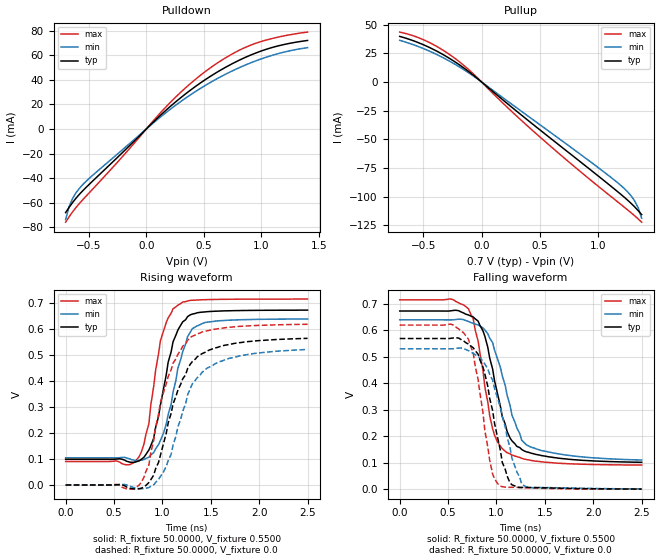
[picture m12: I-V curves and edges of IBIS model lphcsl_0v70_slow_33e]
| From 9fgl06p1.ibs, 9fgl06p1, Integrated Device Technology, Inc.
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[Model]   lphcsl_0v70_slow_33e
Model_type Output
Polarity   Inverting
Enable   Active-High
Vmeas =  0.4000V
Cref =   2.0000pF
Rref =   0.0
Vref =   0.4000V
C_comp   1.1000pF   1.0000pF   1.2000pF
[Temperature Range]   25.0000   85.0000   -40.0000
[Voltage Range]   0.7000V   0.6700V   0.7400V
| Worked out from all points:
|   slope of the pulldown table from 0 to 0.105 V, typ, clamps not added: 10.9 ohm
|   slope of the pullup table from 0 to 0.105 V, typ, clamps not added: 11.6 ohm
|   rising waveform, R_fixture 50.0000, V_fixture 0.5500: 20-80 % time 192ps typ, 209ps min, 165ps max; typ from 0.099 V to 0.672 V
|   rising waveform, R_fixture 50.0000, V_fixture 0.0: 20-80 % time 288ps typ, 300ps min, 271ps max; typ from 0 V to 0.563 V
|   falling waveform, R_fixture 50.0000, V_fixture 0.5500: 20-80 % time 218ps typ, 259ps min, 183ps max; typ from 0.672 V to 0.102 V
|   falling waveform, R_fixture 50.0000, V_fixture 0.0: 20-80 % time 190ps typ, 227ps min, 157ps max; typ from 0.568 V to 0.001 V
[Pulldown]
|Voltage   I(typ)   I(min)   I(max)
-700mV    -68.01mA   -73.7mA    -75.8mA
-670mV    -63.71mA   -63.29mA   -71.42mA
-640mV    -59.83mA   -56.58mA   -67.45mA
-580mV    -53.07mA   -48.2mA    -60.55mA
-520mV    -47.27mA   -42.3mA    -54.39mA
170mV     15.18mA    13.27mA    17.9mA
320mV     27.03mA    23.73mA    31.72mA
470mV     37.47mA    33.03mA    43.69mA
680mV     49.79mA    44.19mA    57.46mA
890mV     59.52mA    53.22mA    67.62mA
1.13V     67.27mA    60.95mA    74.47mA
1.4V      72.06mA    66.21mA    78.86mA
[Pullup]
|Voltage   I(typ)   I(min)   I(max)
-700mV    39.71mA    36.3mA     43.49mA
-580mV    35.81mA    32.37mA    40.12mA
-460mV    30.74mA    27.51mA    35.06mA
-220mV    17.02mA    14.97mA    19.97mA
-70mV     5.896mA    5.136mA    7.022mA
350mV     -29.63mA   -26.26mA   -34.41mA
770mV     -63.63mA   -57.46mA   -71.78mA
1.1V      -90.4mA    -82.71mA   -99.38mA
1.25V     -103.2mA   -95.91mA   -111.7mA
1.31V     -109mA     -103.8mA   -116.8mA
1.34V     -112.3mA   -109.8mA   -119.5mA
1.37V     -115.8mA   -118.9mA   -122.4mA
[Ramp]
| variable   typ   min   max
dV/dt_r  0.3379/0.2954n   0.3123/0.3248n   0.3703/0.2635n
dV/dt_f  0.3418/0.2381n   0.3163/0.2687n   0.3737/0.1983n
R_load = 50.0000
[Rising Waveform]
R_fixture= 50.0000
V_fixture= 0.5500
V_fixture_min= 0.5200
V_fixture_max= 0.5800
|time   V(typ)   V(min)   V(max)
0s        98.56mV    104.2mV    90.22mV
660ps     88.18mV    100.7mV    78.13mV
760ps     92.78mV    94.19mV    109.3mV
860ps     134mV      106.6mV    234.8mV
980ps     307.9mV    171.6mV    554.8mV
1.06ns    472.2mV    271.4mV    642.1mV
1.16ns    595.2mV    449.4mV    690.7mV
1.26ns    646.7mV    569.6mV    706.7mV
1.41ns    663.9mV    619.8mV    711.5mV
2.5ns     671.6mV    637.7mV    714.1mV
[Rising Waveform]
R_fixture= 50.0000
V_fixture= 0.0
V_fixture_min= 0.0
V_fixture_max= 0.0
|time   V(typ)   V(min)   V(max)
0s        0V         0V         0V
760ps     -14.65mV   -13.93mV   62.88uV
860ps     9.248mV    -10.24mV   76.78mV
960ps     86.84mV    21.5mV     271.9mV
1.01ns    157mV      49.52mV    353.9mV
1.11ns    311.2mV    152.8mV    467.7mV
1.29ns    465mV      371.7mV    567.4mV
1.44ns    509.4mV    442.8mV    589.9mV
1.69ns    540mV      486.5mV    605.8mV
2.5ns     563.2mV    520.5mV    617.2mV
[Falling Waveform]
R_fixture= 50.0000
V_fixture= 0.5500
V_fixture_min= 0.5200
V_fixture_max= 0.5800
|time   V(typ)   V(min)   V(max)
0s        672mV      638.7mV    714.2mV
530ps     672.9mV    638.5mV    717.1mV
710ps     657.1mV    632.8mV    680.6mV
760ps     649.5mV    625.8mV    642.1mV
860ps     597.3mV    608.3mV    448.2mV
960ps     453.3mV    553mV      228.4mV
1.11ns    217.4mV    354.2mV    137.6mV
1.26ns    150.1mV    185.2mV    116.4mV
1.34ns    138.3mV    161.4mV    110.1mV
2.5ns     101.6mV    110mV      91.1mV
[Falling Waveform]
R_fixture= 50.0000
V_fixture= 0.0
V_fixture_min= 0.0
V_fixture_max= 0.0
|time   V(typ)   V(min)   V(max)
0s        568.3mV    529.7mV    619mV
530ps     569.2mV    529.5mV    622.3mV
710ps     547.4mV    522.6mV    565.9mV
760ps     533.5mV    512.5mV    513.4mV
860ps     460.8mV    483.6mV    290.2mV
960ps     296.6mV    411.5mV    57.66mV
1.04ns    146.6mV    309mV      11.55mV
1.14ns    23.98mV    156.1mV    7.027mV
1.29ns    6.832mV    12.24mV    5.546mV
2.5ns     615.7uV    1.173mV    235.3uV
